(* Logix 5000 Rung export; software revision 16.00 *)

TYPE BC3GM_SMS_Write :   // SMS data written to BC-3GM
STRUCT
   Message_Byte_Count : INT;   // Number of bytes in the Output String (Max 160 bytes)
   Message : SINT[160];   // Message to be transmitted (Max 160 Bytes)
   Phone_Count : INT;   // Number of phone numbers that the SMS will be sent to
   Phone_Number_1 : SINT[24];   // full number including prefixes country code (example +16613334455)
   Phone_Number_2 : SINT[24];   // full number including prefixes country code
   Phone_Number_3 : SINT[24];   // full number including prefixes country code
   Phone_Number_4 : SINT[24];   // full number including prefixes country code
   Phone_Number_5 : SINT[24];   // full number including prefixes country code
END_STRUCT
END_TYPE

TYPE BC3GM_CONTROL :   // Contains trigger bits for the functions supported by the BC-3GM. Bit should be set as 1 to trigger request and AOI will automa
STRUCT
   Get_Status : BOOL;   // Reads status data from BC-3GM
   Reset_Status : BOOL;   // Resets status counters from BC-3GM
   Write_SMS : BOOL;   // Sends SMS message to BC-3GM
   Read_SMS : BOOL;   // Reads SMS message from BC-3GM
END_STRUCT
END_TYPE

TYPE BC3GM_SMS :   // Stores main SMS functions
STRUCT
   READ : BC3GM_SMS_Read;   // Reads SMS data from BC-3GM
   WRITE : BC3GM_SMS_Write;   // Writes SMS message to BC-3GM
END_STRUCT
END_TYPE

TYPE BC3GM_SMS_Read :   // SMS data read from BC-3GM
STRUCT
   Date_Time : SINT[32];   // The date time to receive SMS text
   Phone_Number : SINT[24];   // full number including prefixes country code etc..
   Message : SINT[160];   // Received the message text
END_STRUCT
END_TYPE

TYPE BC3GM_ModuleDef :   // Main BC-3GM definition
STRUCT
   CONTROL : BC3GM_CONTROL;   // Trigger bits used to request functions from BC-3GM
   STATUS : BC3GM_STATUS;   // BC-3GM status
   SMS : BC3GM_SMS;   // SMS send and receive functions
   UTIL : BC3GM_UTIL;   // Tags used for internal processing - do not update the values
END_STRUCT
END_TYPE

TYPE BC3GM_UTIL :   // Internal tag used for internal ladder processing. Not to be updated by user application
STRUCT
   Status : SINT[140];
   SMS : SINT[284];
   ResetStatus : SINT;
   Test_SMS_Rx_Phone : BOOL;
   Test_SMS_Rx_Text : BOOL;
   Test_SMS_Rx_Time : BOOL;
END_STRUCT
END_TYPE

TYPE BC3GM_STATUS :   // BC-3GM Status
STRUCT
   RSSI : SINT;   // Current Signal Strength dBm
   Min_RSSI : SINT;   // Signal Strength Minimum(since power on)
   Max_RSSI : SINT;   // Signal Strength Maximum(since power on)
   Cell_Net_State : SINT;   // Status of the connection to the Cellular Network
   MAC : SINT[6];   // MAC ID of BC-3GM
   WAN_IP : INT[4];   // Cellular network IP
   RESERVED1 : SINT;
   RESERVED2 : SINT;
   RESERVED3 : INT;
   RESERVED4 : INT;
   Cell_Net_Disconnects : DINT;   // Number of times Modem is disconnected from the cellular network since power on
   LAN_KBytes_Sent : DINT;   // Number Kbytes sent on LAN since power on
   LAN_KBytes_Received : DINT;   // Number of Kbytes received LAN since power on
   WAN_Bytes_Sent : DINT;   // Number of Bytes Sent WAN since power on
   WAN_Bytes_Received : DINT;   // Number of bytes received WAN since power on
   SMS_MSGs_Sent : DINT;   // Number of SMS Messages Sent since power on
   SMS_MSGs_Received : DINT;   // Number of SMS Messages Sent since power on
   PowerOnTime_Year : INT;   // Power on time year
   PowerOnTime_Month : INT;   // Power on time month
   PowerOnTime_Day : INT;   // Power on time day
   PowerOnTime_Hour : INT;   // Power on time hour
   PowerOnTime_Minute : INT;   // Power on time minute
   PowerOnTime_Second : INT;   // Power on time second
   Link_Time_Day : INT;   // Link time day
   Link_Time_Hour : DINT;   // Link time hour
   Link_Time_Minute : INT;   // Link time minute
   Link_Time_Second : INT;   // Link time second
   Temperature_Current : REAL;   // Current temperature
   Temperature_Min : REAL;   // Min temperature
   Temperature_Max : REAL;   // Max temperature
   Data_Usage_Current_Day : DINT;   // Data usage of today
   Data_Usage_Current_Month : DINT;   // Data usage of current month
   Data_Usage_Previous_Day : DINT;   // Data usage of yesterday
   Data_Usage_Previous_Month : DINT;   // Data usage of last month
   FW_Version : REAL;   // Firmware Version of the unit
   Phone_Number : SINT[18];   // Cellular phone number
   IMEI : SINT[20];   // IMEI number
   RESERVED5 : SINT[2];
END_STRUCT
END_TYPE

ADD_ON_INSTRUCTION AOI_BC3GM   (* revision 1.1, vendor Beacon Global Technology Inc. *)
// Add-On Instruction for BC-3GM Industrial Cellular Gateway
// Revision note:
// 1.0     03/20/15    Release
VAR_IN_OUT
   BC3GM : BC3GM_ModuleDef; {required}
   BC3GM_MSG_GET_STATUS : MESSAGE; {required}
   BC3GM_MSG_READ_SMS_PHONE : MESSAGE; {required}
   BC3GM_MSG_READ_SMS_TEXT : MESSAGE; {required}
   BC3GM_MSG_READ_SMS_TIME : MESSAGE; {required}
   BC3GM_MSG_RESET_STATUS : MESSAGE; {required}
   BC3GM_MSG_WRITE_SMS : MESSAGE; {required}
END_VAR

ROUTINE Logic   (* ladder *)
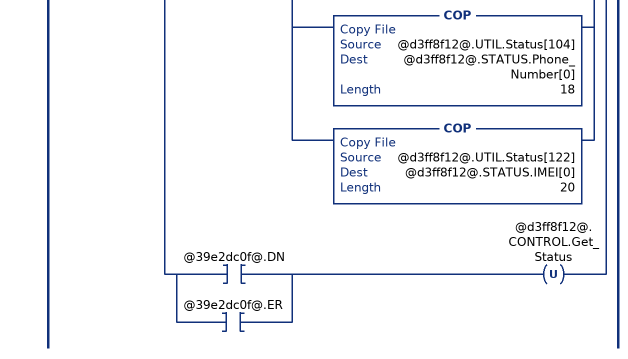
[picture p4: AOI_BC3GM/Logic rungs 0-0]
   0: XIC(@d3ff8f12@.CONTROL.Get_Status)[MSG(@39e2dc0f@) ,XIC(@39e2dc0f@.DN) [COP(@d3ff8f12@.UTIL.Status[0],@d3ff8f12@.STATUS.RSSI,4) ,COP(@d3ff8f12@.UTIL.Status[4],@d3ff8f12@.STATUS.MAC[0],6) ,MVM(0,65280,@d3ff8f12@.STATUS.WAN_IP[0]) ,MVM(@d3ff8f12@.UTIL.Status[10],255,@d3ff8f12@.STATUS.WAN_IP[0]) ,MVM(0,65280,@d3ff8f12@.STATUS.WAN_IP[1]) ,MVM(@d3ff8f12@.UTIL.Status[11],255,@d3ff8f12@.STATUS.WAN_IP[1]) ,MVM(0,65280,@d3ff8f12@.STATUS.WAN_IP[2]) ,MVM(@d3ff8f12@.UTIL.Status[12],255,@d3ff8f12@.STATUS.WAN_IP[2]) ,MVM(0,65280,@d3ff8f12@.STATUS.WAN_IP[3]) ,MVM(@d3ff8f12@.UTIL.Status[13],255,@d3ff8f12@.STATUS.WAN_IP[3]) ,COP(@d3ff8f12@.UTIL.Status[20],@d3ff8f12@.STATUS.Cell_Net_Disconnects,1) ,COP(@d3ff8f12@.UTIL.Status[24],@d3ff8f12@.STATUS.LAN_KBytes_Sent,1) ,COP(@d3ff8f12@.UTIL.Status[28],@d3ff8f12@.STATUS.LAN_KBytes_Received,1) ,COP(@d3ff8f12@.UTIL.Status[32],@d3ff8f12@.STATUS.WAN_Bytes_Sent,1) ,COP(@d3ff8f12@.UTIL.Status[36],@d3ff8f12@.STATUS.WAN_Bytes_Received,1) ,COP(@d3ff8f12@.UTIL.Status[40],@d3ff8f12@.STATUS.SMS_MSGs_Sent,1) ,COP(@d3ff8f12@.UTIL.Status[44],@d3ff8f12@.STATUS.SMS_MSGs_Received,1) ,COP(@d3ff8f12@.UTIL.Status[48],@d3ff8f12@.STATUS.PowerOnTime_Year,1) ,COP(@d3ff8f12@.UTIL.Status[50],@d3ff8f12@.STATUS.PowerOnTime_Month,1) ,COP(@d3ff8f12@.UTIL.Status[52],@d3ff8f12@.STATUS.PowerOnTime_Day,1) ,COP(@d3ff8f12@.UTIL.Status[54],@d3ff8f12@.STATUS.PowerOnTime_Hour,1) ,COP(@d3ff8f12@.UTIL.Status[56],@d3ff8f12@.STATUS.PowerOnTime_Minute,1) ,COP(@d3ff8f12@.UTIL.Status[58],@d3ff8f12@.STATUS.PowerOnTime_Second,1) ,COP(@d3ff8f12@.UTIL.Status[60],@d3ff8f12@.STATUS.Link_Time_Day,1) ,COP(@d3ff8f12@.UTIL.Status[64],@d3ff8f12@.STATUS.Link_Time_Hour,1) ,COP(@d3ff8f12@.UTIL.Status[68],@d3ff8f12@.STATUS.Link_Time_Minute,1) ,COP(@d3ff8f12@.UTIL.Status[70],@d3ff8f12@.STATUS.Link_Time_Second,1) ,COP(@d3ff8f12@.UTIL.Status[72],@d3ff8f12@.STATUS.Temperature_Current,1) ,COP(@d3ff8f12@.UTIL.Status[76],@d3ff8f12@.STATUS.Temperature_Min,1) ,COP(@d3ff8f12@.UTIL.Status[80],@d3ff8f12@.STATUS.Temperature_Max,1) ,COP(@d3ff8f12@.UTIL.Status[84],@d3ff8f12@.STATUS.Data_Usage_Current_Day,1) ,COP(@d3ff8f12@.UTIL.Status[88],@d3ff8f12@.STATUS.Data_Usage_Current_Month,1) ,COP(@d3ff8f12@.UTIL.Status[92],@d3ff8f12@.STATUS.Data_Usage_Previous_Day,1) ,COP(@d3ff8f12@.UTIL.Status[96],@d3ff8f12@.STATUS.Data_Usage_Previous_Month,1) ,COP(@d3ff8f12@.UTIL.Status[100],@d3ff8f12@.STATUS.FW_Version,1) ,COP(@d3ff8f12@.UTIL.Status[104],@d3ff8f12@.STATUS.Phone_Number[0],18) ,COP(@d3ff8f12@.UTIL.Status[122],@d3ff8f12@.STATUS.IMEI[0],20) ] ,[XIC(@39e2dc0f@.DN) ,XIC(@39e2dc0f@.ER) ] OTU(@d3ff8f12@.CONTROL.Get_Status) ];
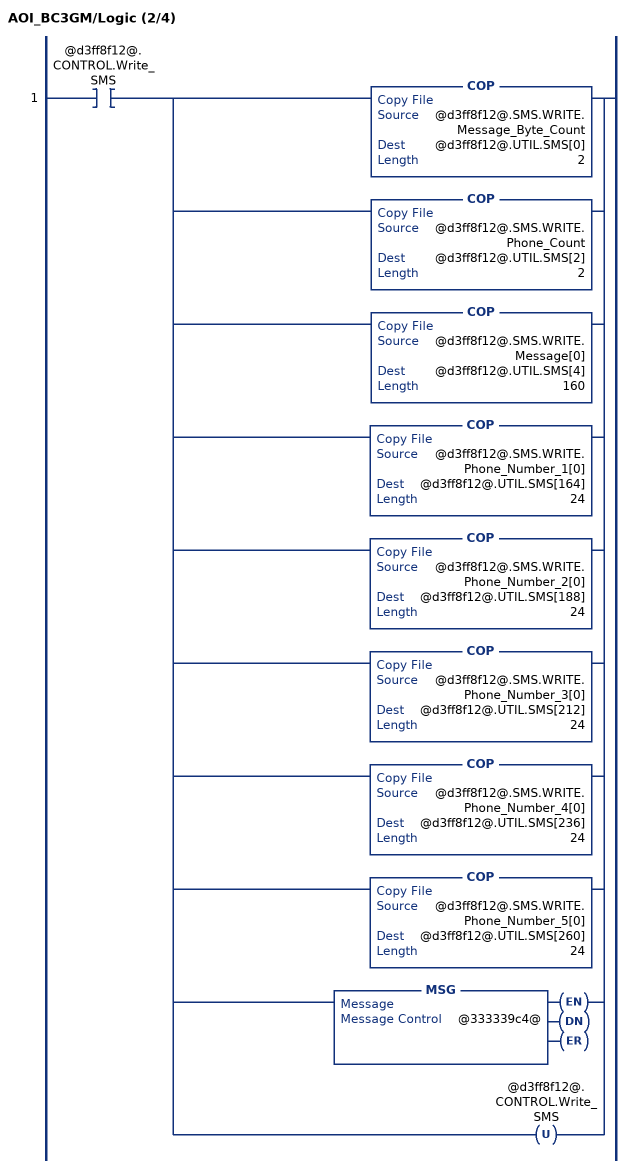
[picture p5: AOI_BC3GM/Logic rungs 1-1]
   1: XIC(@d3ff8f12@.CONTROL.Write_SMS)[COP(@d3ff8f12@.SMS.WRITE.Message_Byte_Count,@d3ff8f12@.UTIL.SMS[0],2) ,COP(@d3ff8f12@.SMS.WRITE.Phone_Count,@d3ff8f12@.UTIL.SMS[2],2) ,COP(@d3ff8f12@.SMS.WRITE.Message[0],@d3ff8f12@.UTIL.SMS[4],160) ,COP(@d3ff8f12@.SMS.WRITE.Phone_Number_1[0],@d3ff8f12@.UTIL.SMS[164],24) ,COP(@d3ff8f12@.SMS.WRITE.Phone_Number_2[0],@d3ff8f12@.UTIL.SMS[188],24) ,COP(@d3ff8f12@.SMS.WRITE.Phone_Number_3[0],@d3ff8f12@.UTIL.SMS[212],24) ,COP(@d3ff8f12@.SMS.WRITE.Phone_Number_4[0],@d3ff8f12@.UTIL.SMS[236],24) ,COP(@d3ff8f12@.SMS.WRITE.Phone_Number_5[0],@d3ff8f12@.UTIL.SMS[260],24) ,MSG(@333339c4@) ,OTU(@d3ff8f12@.CONTROL.Write_SMS) ];
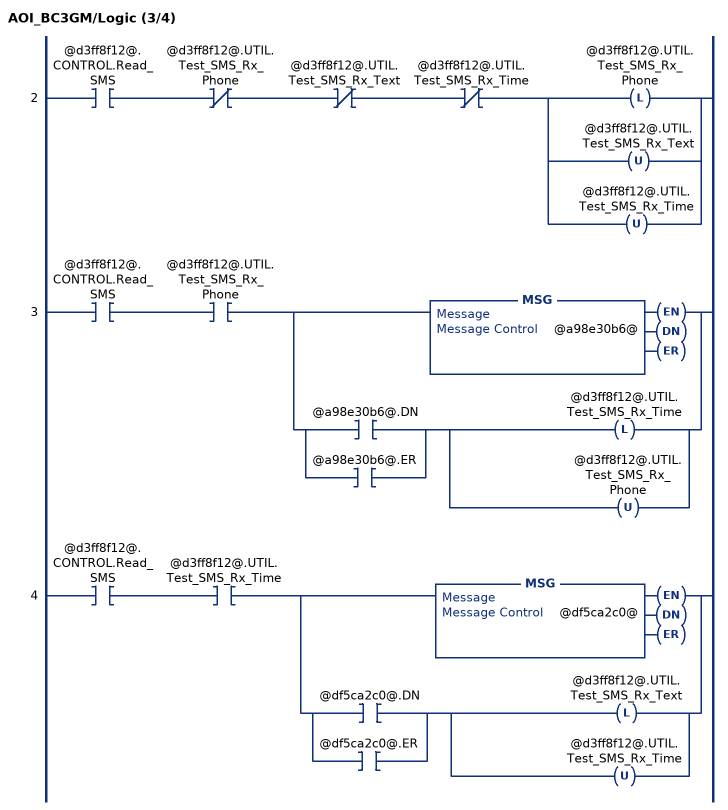
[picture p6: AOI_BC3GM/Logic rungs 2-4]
   2: XIC(@d3ff8f12@.CONTROL.Read_SMS)XIO(@d3ff8f12@.UTIL.Test_SMS_Rx_Phone)XIO(@d3ff8f12@.UTIL.Test_SMS_Rx_Text)XIO(@d3ff8f12@.UTIL.Test_SMS_Rx_Time)[OTL(@d3ff8f12@.UTIL.Test_SMS_Rx_Phone) ,OTU(@d3ff8f12@.UTIL.Test_SMS_Rx_Text) ,OTU(@d3ff8f12@.UTIL.Test_SMS_Rx_Time) ];
   3: XIC(@d3ff8f12@.CONTROL.Read_SMS)XIC(@d3ff8f12@.UTIL.Test_SMS_Rx_Phone)[MSG(@a98e30b6@) ,[XIC(@a98e30b6@.DN) ,XIC(@a98e30b6@.ER) ] [OTL(@d3ff8f12@.UTIL.Test_SMS_Rx_Time) ,OTU(@d3ff8f12@.UTIL.Test_SMS_Rx_Phone) ] ];
   4: XIC(@d3ff8f12@.CONTROL.Read_SMS)XIC(@d3ff8f12@.UTIL.Test_SMS_Rx_Time)[MSG(@df5ca2c0@) ,[XIC(@df5ca2c0@.DN) ,XIC(@df5ca2c0@.ER) ] [OTL(@d3ff8f12@.UTIL.Test_SMS_Rx_Text) ,OTU(@d3ff8f12@.UTIL.Test_SMS_Rx_Time) ] ];
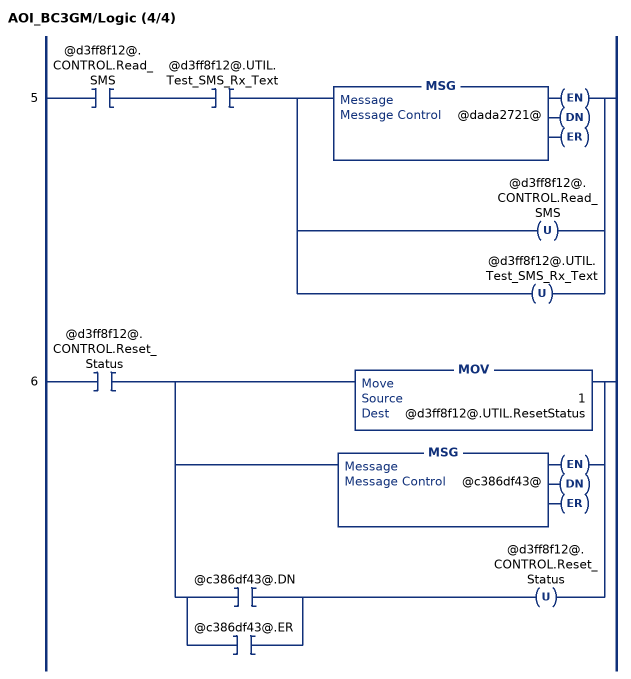
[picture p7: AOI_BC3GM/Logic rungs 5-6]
   5: XIC(@d3ff8f12@.CONTROL.Read_SMS)XIC(@d3ff8f12@.UTIL.Test_SMS_Rx_Text)[MSG(@dada2721@) ,OTU(@d3ff8f12@.CONTROL.Read_SMS) ,OTU(@d3ff8f12@.UTIL.Test_SMS_Rx_Text) ];
   6: XIC(@d3ff8f12@.CONTROL.Reset_Status)[MOV(1,@d3ff8f12@.UTIL.ResetStatus) ,MSG(@c386df43@) ,[XIC(@c386df43@.DN) ,XIC(@c386df43@.ER) ] OTU(@d3ff8f12@.CONTROL.Reset_Status) ];
END_ROUTINE
END_ADD_ON_INSTRUCTION

VAR_GLOBAL   (* controller tags *)
   BC3GM : BC3GM_ModuleDef;
   BC3GM_MSG_WRITE_SMS : MESSAGE;
        MessageParameters(MessageType := CIP Generic, RequestedLength := 284, ConnectedFlag := 2, ServiceCode := 16#0002, ObjectType := 16#00a4, TargetObject := 1, LocalElement := BC3GM.UTIL.SMS[0], DestinationTag := BC3GM)
   AOI_BC3GM : AOI_BC3GM;
   BC3GM_MSG_GET_STATUS : MESSAGE;
        MessageParameters(MessageType := CIP Generic, RequestedLength := 142, ConnectedFlag := 2, ServiceCode := 16#0001, ObjectType := 16#00a1, TargetObject := 1, LocalElement := BC3GM, DestinationTag := BC3GM.UTIL.Status[0])
   BC3GM_MSG_READ_SMS_TIME : MESSAGE;
        MessageParameters(MessageType := CIP Data Table Read, RemoteElement := RX_SMS_TEXT.DateTime, RequestedLength := 32, ConnectedFlag := 2, LocalElement := BC3GM.SMS.READ.Date_Time[0])
   BC3GM_MSG_READ_SMS_TEXT : MESSAGE;
        MessageParameters(MessageType := CIP Data Table Read, RemoteElement := RX_SMS_TEXT.Text_Str, RequestedLength := 160, ConnectedFlag := 2, LocalElement := BC3GM.SMS.READ.Message[0])
   BC3GM_MSG_RESET_STATUS : MESSAGE;
        MessageParameters(MessageType := CIP Generic, RequestedLength := 1, ConnectedFlag := 2, ServiceCode := 16#0010, ObjectType := 16#00a2, TargetObject := 1, AttributeNumber := 16#0001, LocalElement := BC3GM.UTIL.ResetStatus)
   BC3GM_MSG_READ_SMS_PHONE : MESSAGE;
        MessageParameters(MessageType := CIP Data Table Read, RemoteElement := RX_SMS_TEXT.Phone_Number, RequestedLength := 24, ConnectedFlag := 2, LocalElement := BC3GM.SMS.READ.Phone_Number[0])
END_VAR

PROGRAM MainProgram

ROUTINE MainRoutine   (* ladder *)
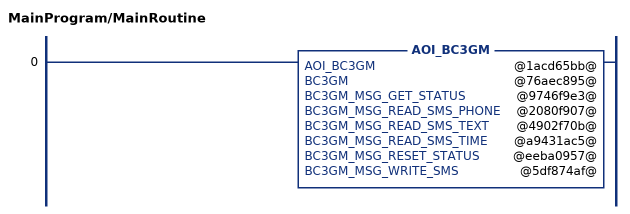
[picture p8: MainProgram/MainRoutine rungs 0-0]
   0: AOI_BC3GM(@1acd65bb@,@76aec895@,@9746f9e3@,@2080f907@,@4902f70b@,@a9431ac5@,@eeba0957@,@5df874af@);
END_ROUTINE
END_PROGRAM
